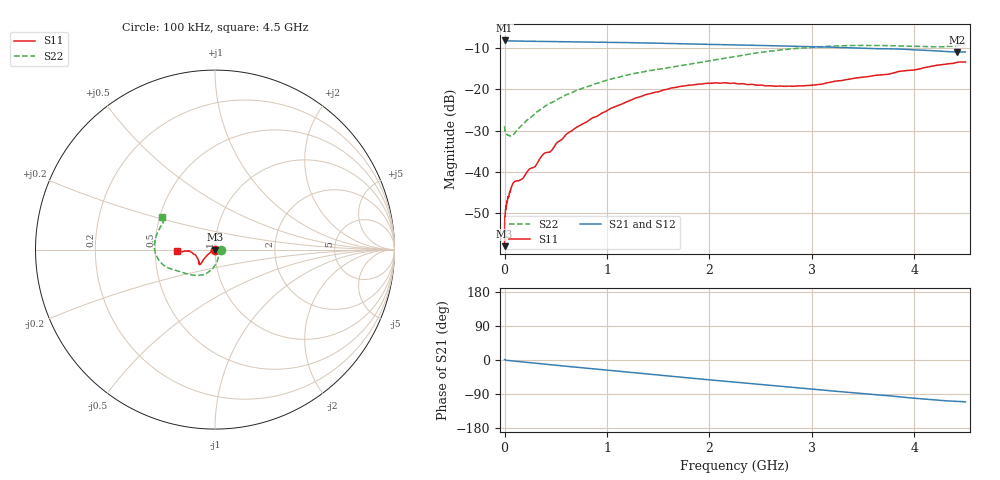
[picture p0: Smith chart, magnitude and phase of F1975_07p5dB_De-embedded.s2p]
! Integrated Device Technology
! Corporate Headquarters
! 6024 Silver Creek Valley Road
! San Jose, CA 95138  USA
! Phone:  1-408-284-8200
! Toll Free:  1-800-223-1366
! Webpage:  http://www.idt.com/
! Timing and RF Division
! 515 Groton Road, Suite 102
! Westford, MA 01886-6024
! Device:  F1975
! Description: 6-bit, 75 ohm, 0.5 dB Digital Step Attenuator
! Frequency:  5.0 MHz -  3.00 GHz
! Package:  4x4 mm QFN Plastic Package: 20 pin
! Ports:  2 RF, 11 DC
!  Pin  1  = D5 (16 dB)
!  Pin  2  = RF1  =  Port 1
!  Pin  3  = Serial Data In (DATA)
!  Pin  4  = Serial Clock (CLK)
!  Pin  5  = Serial Latch Enable (LE)
!  Pin  6  = VDD
!  Pin  7  = NC
!  Pin  8  = NC
!  Pin  9  = NC
!  Pin 10  = GND
!  Pin 11  = GND
!  Pin 12  = NC
!  Pin 13  = VMODE
!  Pin 14  = RF2  =  Port 2
!  Pin 15  = D4 (8 dB)
!  Pin 16  = D3 (4 dB)
!  Pin 17  = D2 (2 dB)
!  Pin 18  = NC
!  Pin 19  = D1 (1 dB)
!  Pin 20  = D0 (0.5 dB)
! State:  15
! Atten State:  7.5 dB
! Voltage:  +3.30 Volts
! Current:  0.564 mA
! Data:  The device was measured on a F1975 evaluation board which has
!  individual transmission lines to the RF pins.  Data was collected
!  using a calibrated network analyzer.  The evaluation board was
!  de-embedded using Automatic Fixture Removal (AFR).
!  The reference plane is the edge of the package pin.
! Misc:
!  Action Tracker AT0415
! Date Measured:  2018-02-08
! Date:  2018-03-26  MJV
! Note:
!  Integrated Device Technology supplies this data as a sample of measured
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# GHz S dB R 75
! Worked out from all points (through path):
!   291 points, 100 kHz to 4.5 GHz, reference 75 ohm
!   highest |S21| = -8.19 dB at 100 kHz (marker M1); lowest = -11.0 dB at 4.42 GHz (marker M2)
!   group delay of S21, straight-line fit = 69.7 ps
!   lowest |S11| = -58.0 dB at 100 kHz (marker M3), VSWR 1.00, Z = 74.8 + j0.00449 ohm
!   |S11| at or under -10 dB: start of sweep to end of sweep
!   |S22| runs from -31.3 to -9.1 dB; largest |S21 - S12| = 0.00017
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0.0001  -57.96 178.6  -8.19 1.2  -8.19 1.2  -28.93 -0.1
0.0002  -55.85 -175.1  -8.20 1.1  -8.20 1.2  -29.07 -0.7
0.0005  -53.68 -168.5  -8.22 1.1  -8.21 1.1  -29.41 -1.8
0.002  -51.03 -168.0  -8.24 0.8  -8.24 0.8  -29.96 -2.8
0.009  -49.05 -163.2  -8.26 -0.3  -8.26 -0.3  -30.50 -7.7
0.032  -46.20 -162.4  -8.29 -1.2  -8.29 -1.2  -31.05 -16.9
0.08  -42.79 -152.6  -8.32 -2.5  -8.32 -2.5  -31.13 -35.3
0.18  -41.55 -146.3  -8.37 -5.3  -8.36 -5.3  -28.41 -56.8
0.24  -39.34 -145.8  -8.39 -6.9  -8.38 -6.9  -27.15 -64.6
0.3  -38.64 -147.9  -8.40 -8.5  -8.40 -8.5  -25.86 -71.3
0.36  -36.22 -149.2  -8.42 -10.1  -8.42 -10.1  -24.67 -75.3
0.46  -34.81 -150.0  -8.45 -12.7  -8.45 -12.7  -23.20 -81.6
0.62  -30.55 -148.8  -8.50 -16.9  -8.50 -16.9  -21.16 -89.5
0.76  -28.42 -145.8  -8.54 -20.6  -8.54 -20.6  -19.76 -96.0
1.04  -24.59 -142.8  -8.64 -28.1  -8.64 -28.1  -17.53 -107.0
1.52  -20.48 -136.5  -8.86 -40.4  -8.86 -40.4  -15.10 -125.2
1.88  -18.78 -135.1  -9.08 -49.4  -9.08 -49.4  -13.60 -139.9
2.26  -18.61 -138.4  -9.28 -58.6  -9.27 -58.6  -12.03 -152.6
3.02  -18.99 -164.1  -9.72 -77.1  -9.71 -77.1  -9.83 -171.4
3.76  -16.29 -176.7  -10.22 -94.5  -10.21 -94.5  -9.47 166.9
4.42  -13.49 -176.3  -11.00 -109.2  -10.99 -109.2  -9.38 149.9
4.5  -13.39 -178.4  -10.97 -110.5  -10.96 -110.5  -9.15 148.5
